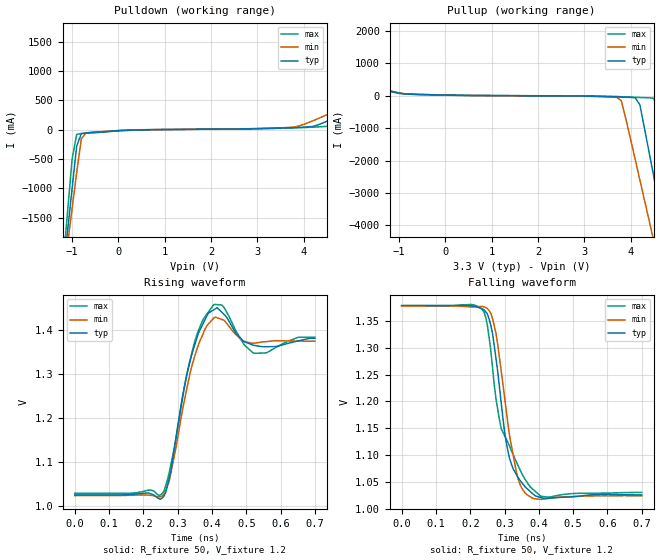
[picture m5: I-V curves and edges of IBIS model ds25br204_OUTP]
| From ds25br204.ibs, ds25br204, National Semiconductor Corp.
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[Model]   ds25br204_OUTP
Model_type Output
Polarity Non-Inverting
Vref=1.2
Vmeas=1.2
Rref=50   | 100 Ohms Across Outputs OUTP and OUTN
Cref=0p
C_comp   1.2pF   1.2pF   1.2pF
[Temperature Range]   25   85   -40
[Voltage Range]   3.3   3.0   3.6
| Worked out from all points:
|   slope of the pulldown table from 0 to 0.495 V, typ, clamps not added: 34.1 ohm
|   slope of the pullup table from 0 to 0.495 V, typ, clamps not added: 46.6 ohm
|   rising waveform, R_fixture 50, V_fixture 1.2: 20-80 % time 47ps typ, 51.8ps min, 48.4ps max; typ from 1.02 V to 1.38 V
|   falling waveform, R_fixture 50, V_fixture 1.2: 20-80 % time 44.7ps typ, 46.9ps min, 68.4ps max; typ from 1.38 V to 1.03 V
[Pullup]
|Vtable   I(typ)   I(min)   I(max)
-3.6V     2.054A     2.034A     2.086A
-2.8V     982.7mA    1.113A     894.6mA
-2.3V     586.9mA    582.3mA    612.2mA
-1V       80.49mA    89.94mA    71.24mA
3.7V      -38.65mA   -52.47mA   -26.27mA
3.8V      -43.53mA   -153.8mA   -32.69mA
4.2V      -278.7mA   -2.593A    -54.97mA
4.5V      -2.487A    -4.473A    -78.69mA
4.6V      -3.229A    -5.1A      -507.7mA
4.7V      -3.972A    -5.726A    -1.428A
5V        -6.198A    -7.605A    -4.211A
7.2V      -22.47A    -21.34A    -24.57A
[Pulldown]
|V(pulldown)   I(typ)   I(min)   I(max)
-3.6V     -20.29A    -17.64A    -24.61A
-1.2V     -2.491A    -2.602A    -2.354A
-1.1V     -1.75A     -1.975A    -1.428A
-1V       -1.011A    -1.35A     -507.3mA
-900mV    -280.1mA   -728.1mA   -78.43mA
-800mV    -66.5mA    -157.2mA   -64.76mA
-700mV    -54.24mA   -54.89mA   -59.61mA
3.7V      33.65mA    40.46mA    29.43mA
4.7V      218.5mA    327.7mA    100mA
5.9V      761.4mA    1.238A     618.1mA
6.4V      1.397A     1.817A     905.8mA
7.2V      2.476A     2.747A     2.104A
[Ramp]
|   typ   min   max
dV/dt_r   212m/36p   201m/43p   219m/37p
dV/dt_f   212m/36p   201m/43p   219m/37p
R_load=50
[Rising Waveform]
R_fixture=50
V_fixture=1.2
V_fixture_min=1.1997
V_fixture_max=1.2026
0s        1.025V     1.024V     1.029V
260ps     1.022V     1.026V     1.034V
280ps     1.079V     1.073V     1.093V
315ps     1.252V     1.222V     1.248V
340ps     1.341V     1.313V     1.344V
370ps     1.408V     1.384V     1.416V
405ps     1.445V     1.427V     1.457V
435ps     1.435V     1.422V     1.451V
520ps     1.365V     1.369V     1.347V
700ps     1.381V     1.374V     1.383V
[Falling Waveform]
R_fixture=50
V_fixture=1.2
V_fixture_min=1.1997
V_fixture_max=1.2026
0s        1.379V     1.377V     1.378V
215ps     1.377V     1.376V     1.379V
240ps     1.371V     1.376V     1.367V
255ps     1.353V     1.369V     1.319V
285ps     1.227V     1.282V     1.167V
310ps     1.107V     1.157V     1.123V
335ps     1.063V     1.066V     1.086V
365ps     1.038V     1.026V     1.05V
425ps     1.019V     1.019V     1.022V
700ps     1.026V     1.024V     1.03V
